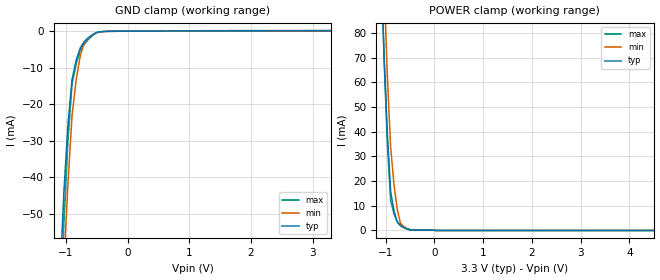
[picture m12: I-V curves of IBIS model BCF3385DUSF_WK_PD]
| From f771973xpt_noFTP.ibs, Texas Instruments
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|   Model Cell BCF3385DUSF_WK_PD
|BCF3385DUSF_WK_PD
[Model]   BCF3385DUSF_WK_PD
Model_type   Input
Polarity   Non-Inverting
Vinl =  0.8
Vinh =  2
C_comp   1.190763p   1.060544p   1.317111p
[Model Spec]
Vinl   0.8   0.8   0.8
Vinh   2   2   2
[Temperature Range]   25   155   -40
[Voltage Range]   3.3   2.97   3.63
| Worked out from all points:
|   GND clamp passes 1 mA (typ) near -0.57 V on its own axis
|   POWER clamp passes 1 mA (typ) near -0.61 V on its own axis
| Nom Voltages:
|   VDD=1.2, VDDS=3.3, VSS=0
| Min Voltages:
|   VDD=1.08, VDDS=2.97, VSS=0
| Max Voltages:
|   VDD=1.32, VDDS=3.63, VSS=0
[POWER_clamp]
|   voltage   I(typ)   I(min)   I(max)
-3.3V     1.919A     2.431A     2.07A
-1.1V     109.6mA    140.7mA    112.7mA
-1.033V   69.94mA    97.96mA    68.83mA
-966.7mV  38.68mA    62.26mA    35.3mA
-900mV    15.79mA    33.62mA    12.12mA
-833.3mV  8.093mA    18.99mA    6.86mA
-766.7mV  3.45mA     8.781mA    3.617mA
-700mV    1.863mA    2.994mA    2.393mA
-633.3mV  1.154mA    1.592mA    1.5mA
-500mV    241.1uA    272.1uA    323.7uA
-300mV    107.7uA    54.49uA    178.9uA
6.6V      0A         0A         0A
[GND_clamp]
|   voltage   I(typ)   I(min)   I(max)
-3.3V     -1.48A     -1.41A     -2.186A
-1.1V     -69.73mA   -89.96mA   -82.83mA
-1.033V   -44.47mA   -64.24mA   -52.88mA
-966.7mV  -25.63mA   -41.94mA   -30.08mA
-900mV    -13.22mA   -23.06mA   -14.42mA
-833.3mV  -8.012mA   -13.34mA   -8.913mA
-766.7mV  -4.54mA    -6.685mA   -5.281mA
-700mV    -2.798mA   -3.107mA   -3.521mA
-566.7mV  -921.2uA   -975.4uA   -1.153mA
-500mV    -307.5uA   -405.6uA   -363.2uA
-300mV    -27.98uA   -20.38uA   -40.75uA
3.3V      107.2uA    58.01uA    177.9uA
